{attribute 'no_check'}
//Provides all information of PlcAppSystemInfo plus addtional infos like time stamps from various source and in different formats
//
//PlcAppSystemInfo -> https://infosys.beckhoff.com/english.php?content=../content/1033/globaldatatypes/9007199969559691.html&id=7934476013631172214
//TwimCAT time sources -> https://infosys.beckhoff.com/english.php?content=../content/1033/ethercatsystem/2469114379.html&id=
//
FUNCTION_BLOCK SystemInfo
VAR_OUTPUT CONSTANT
{attribute 'displaymode':='binary'}
	OPTION_US_DATE_FORMAT									:	BYTE := 2#0000_0001; //Enable US date format in time stamp - mm/dd/yy
{attribute 'displaymode':='binary'}
	OPTION_US_TIME_FORMAT									:	BYTE := 2#0000_0010; //Enable time in US format - AM/PM vs 24h
{attribute 'displaymode':='binary'} 
	OPTION_TIME_STR_ADD_MS									:	BYTE := 2#0000_0100; //Add ms to time string 
{attribute 'displaymode':='binary'} 
	OPTION_DISABLE_DEV_IDENT								:	BYTE := 2#0000_1000; //Disable to read device identification during boot up (Call FB_GetDeviceIdentificationEx)
END_VAR                     								
VAR_INPUT                   						
	Enable													:	BOOL := TRUE; //Enable function block
	ResetTrig												:	BOOL := FALSE; //Reset Old boot data fault signal
	RtcSyncCylce											:	DWORD := 60; //in seconds - see documentation for "FB_LocalSystemTime"
	KeepOutputsOnBP 										: 	BOOL := FALSE; //The flag can be set to avoid that the outputs are zero-filled if a breakpoint is reached. The task keeps running. Only the execution of PLC code is interrupted.
{attribute 'displaymode':='binary'}
	Options													:	BYTE := 2#0000_0000; //option constants are alreay predefined, so they can accordingly be passed symbolically to the block 
	DateStrSeperator										:	STRING(1) := '/';
END_VAR
VAR_OUTPUT
//PlcAppSystemInfo and cycle time inforamtion from caller task 
	ObjId													: 	OTCID; //Object ID of the PLC project instance
	AdsPort 												: 	UINT; //ADS port of PLC application 
	TComSrvPtr 												: 	ITComObjectServer; // Pointer to TcCOM Object Server 
	AppName													: 	STRING(63); //TwinCAT generated name containing the port number. 
	ProjectName 											: 	STRING(63); //The name of the PLC project. 
	AppTimestampDT											:	DT; //Date and time of application start 
	AppTimestamp											:	STRING(25);	//Date and time of application start in string format
	TaskIndex												:	INT ; //Task index of SysInfo caller
	TaskCnt													: 	UDINT; //The number of tasks in the actual runtime system
	
	Flags 													: 	DWORD; //Boot flags
	LicensesPending 										: 	BOOL;
	BSODOccured 											: 	BOOL;										
	BootDataLoaded											: 	BOOL;//PERSISTENT variables: LOADED (without error)
	OldBootData												: 	BOOL; //PERSISTENT variables: INVALID (the back-up copy was loaded, since no valid data was present)
	NoBootDataLoaded										:	BOOL; //Error no boot data loaded
//	PersistentStatus 										: 	EPlcPersistentStatus;

	LoggedIn												:	BOOL;
	ShutdownInProgress 										: 	BOOL;	
	OnlineChangeCount										: 	UDINT; //The number of online changes made since the last complete download.
	OnlineChange											:	BOOL; //Online change count changed since last plc cycle

{attribute 'displaymode':='hex'}
	CpuCounter												:	ULINT;
	CycleTime         										: 	UDINT;//Cylce time read from PlcAppSystemInfo in multiples of 100 ns.
	CycleTimeNS         									: 	UDINT;//Cylce time in nanoseconds
	CycleTimeT       										: 	TIME; //Cycle time in time format
	CycleTimeLT       										: 	LTIME; //Cycle time in ltime format
	CycleTimeFloat											:	LREAL;//Cycle time in float format <s.ms>

	DevIdentValid											:	BOOL;
	pDevIdent												:	POINTER TO ST_DeviceIdentificationEx := ADR(InstGetDevIdent.stDevIdent);
	
//General	
	TimezoneId												: 	E_TimeZoneID;
	TimeZoneInfo											:	ST_TimeZoneInformation;
	MonthDays												:	WORD;
	LeapYear												:	BOOL;
	DayOfYear												:	WORD;
	WeekOfYear												:	WORD;
	UtcTimeFT												:	Tc2_Utilities.T_FILETIME; //Current UTC System/TwinCAT time T_FILETIME format, structure representing a 64-bit value with the a number of 100-nanosecond intervals since January 1, 1601 (UTC) (dwLowDateTime : DWORD / dwHighDateTime : DWORD)
//	UtcTimeFT												:	Tc2_Utilities.T_FILETIME64; //Current UTC System/TwinCAT time T_FILETIME format, structure representing a 64-bit value with the a number of 100-nanosecond intervals since January 1, 1601 (UTC) (dwLowDateTime : DWORD / dwHighDateTime : DWORD)
	UtcTimeSTRUCT											:	Tc2_Utilities.TIMESTRUCT; //Current UTC System/TwinCAT time in TIMESTRUCT format
	UtcTimezoneBias											:	DINT;   //Total timezone bias in minutes to UTC 
	TimeDT													:	DATE_AND_TIME;	//Current time in DATE_AND_TIME format: DT#1970-01-01-00:00 -> DT#2106-02-06-06:28:15
//	TimeLDT													:	LDATE_AND_TIME;	//Current time in 64bit LDATE_AND_TIME format: DT#1970-01-01-00:00 -> DT#2262-4-10-23:59:59.99999999
	TimeTOD													:	TOD; //Current time in TOD format, range from TOD#00:00 -> TOD#1193:02:47.295
	TimeFT													:	Tc2_Utilities.T_FILETIME; //Current time in T_FILETIME format, structur representing a 64-bit value with the a number of 100-nanosecond intervals since January 1, 1601 (UTC) (dwLowDateTime : DWORD / dwHighDateTime : DWORD)
//	TimeFT													:	Tc2_Utilities.T_FILETIME64; //Current time in T_FILETIME format, structur representing a 64-bit value with the a number of 100-nanosecond intervals since January 1, 1601 (UTC) (dwLowDateTime : DWORD / dwHighDateTime : DWORD)
	TimeSTRUCT												:	Tc2_Utilities.TIMESTRUCT; //Current time in TIMESTRUCT format
	Datestamp												:	DATE; //D#1970-01-01 -> D#2106-02-06
	DateStr													:	STRING(15);	(* dd.mm.jj or mm.dd.jj *)	
	TimeStr													:	STRING(15);	(* hh:mm:ss.xxx or hh:mm:ss.xxxPM/AM *)
	TimeStamp												:	STRING(25); (* DateStr + TimeStr *)	
	TimeStamp2												:	STRING(25); (* YYYY-MM-DDTHHMMSS for example YYYY-MM-DD_HHMMSS_Name.txt *)
	TimeStamp3												:	STRING(25); (* YYYY-MM-DD-hh:mm:ss.xxx *)
	DateStrISO												:	STRING(15);	(* jj-mm-dd *)
	TimeStrISO												:	STRING(15);	(* hh:mm:ss *)
	TimeStampISO											:	STRING(25);	(* jj-mm-dd'T'hh:mm:ss.xxms *)	
	TimeStampStartup										:	DATE_AND_TIME; //Timestamp of startup
	DCTime													:	Tc2_EtherCAT.T_DCTIME64; //Current TwinCAT distributed clock time in 64-bit T_DCTIME64 format. The smallest unit is a nanosecond.
	DCTimeSTRUCT											:	Tc2_Utilities.TIMESTRUCT;//Current TwinCAT distributed clock time in TIMESTRUCT format
//	SysTimeFT												:	Tc2_Utilities.T_FILETIME64; //Current UTC System/TwinCAT time T_FILETIME format, structure representing a 64-bit value with the a number of 100-nanosecond intervals since January 1, 1601 (UTC) (dwLowDateTime : DWORD / dwHighDateTime : DWORD)
	SysTimeFT												:	Tc2_Utilities.T_FILETIME; //Current UTC System/TwinCAT time T_FILETIME format, structure representing a 64-bit value with the a number of 100-nanosecond intervals since January 1, 1601 (UTC) (dwLowDateTime : DWORD / dwHighDateTime : DWORD)
	SysTimeSTRUCT											:	Tc2_Utilities.TIMESTRUCT; //Current UTC System/TwinCAT time in TIMESTRUCT format
	
END_VAR
VAR
	(* Inst. Get Taskindex *)
	InstGETCURTASKINDEX										: 	GETCURTASKINDEX;
	InstLocalSystemTime										:	FB_LocalSystemTime;
	InstNtSetLocalTime										:	NT_SetLocalTime := (NETID := '', TMOUT := DEFAULT_ADS_TIMEOUT);
	InstTimeZoneInfo										:	FB_GetTimeZoneInformation;
	InstCpuCouter											:	GETCPUCOUNTER;
	InstSystemTime											:	GetSystemTime;
	
	
	InstGetDevIdent											:	FB_GetDeviceIdentificationEx;
	_OnlineChangeCount										: 	UDINT; 
	_sec													:	WORD;
	_hour													:	WORD;
	_day													:	WORD;
	_Init													:	BOOL;
END_VAR

	(* Evaluate the PlcAppSystemInfo and and get sytstem timestamp					*)
	(********************************************************************************)
	
(* Get Current Task Index ************************************************************************)
	IF InstGETCURTASKINDEX.index = 0 then InstGETCURTASKINDEX(index => TaskIndex); END_IF

(* Read System Info Current Task *****************************************************************)	
	(* Get static information and boot error messages *)
	IF TwinCAT_SystemInfoVarList._TaskInfo[InstGETCURTASKINDEX.Index].FirstCycle 
	THEN
		AppTimestampDT										:= TwinCAT_SystemInfoVarList._AppInfo.AppTimestamp;
		AppTimestamp										:= DT_TO_STRING(AppTimestampDT);
		AppTimestamp										:= DELETE(AppTimestamp,3,1);
			
		TaskIndex											:= InstGETCURTASKINDEX.Index;
		TaskCnt 											:= TwinCAT_SystemInfoVarList._AppInfo.TaskCnt;
		
		ObjId												:= TwinCAT_SystemInfoVarList._AppInfo.ObjId;
		AppName												:= TwinCAT_SystemInfoVarList._AppInfo.AppName;	
		ProjectName											:= TwinCAT_SystemInfoVarList._AppInfo.ProjectName;	
		AdsPort												:= TwinCAT_SystemInfoVarList._AppInfo.AdsPort;	
			
		Flags												:= TwinCAT_SystemInfoVarList._AppInfo.Flags;
//		PersistentStatus									:= TwinCAT_SystemInfoVarList._AppInfo.PersistentStatus;
		
		BootDataLoaded										:= TwinCAT_SystemInfoVarList._AppInfo.BootDataLoaded;
		OldBootData											:= TwinCAT_SystemInfoVarList._AppInfo.OldBootData;
		NoBootDataLoaded									:= NOT BootDataLoaded AND NOT OldBootData;
		BSODOccured 										:= TwinCAT_SystemInfoVarList._AppInfo.BSODOccured;
		
		CycleTime         									:= TwinCAT_SystemInfoVarList._TaskInfo[TaskIndex].CycleTime;
		CycleTimeNS         								:= TwinCAT_SystemInfoVarList._TaskInfo[TaskIndex].CycleTime * 100;
		CycleTimeT											:= LREAL_TO_TIME(UDINT_TO_LREAL(CycleTime) * 0.0001 );
		CycleTimeLT											:= TO_LTIME(CycleTimeNS);	
		CycleTimeFloat										:= (UDINT_TO_LREAL(CycleTime) * 0.0001 / 1000.0);	
		
	ELSIF ResetTrig
	THEN
		resetBootInfo();
	ELSIF NOT Enable
	THEN
		RETURN;
	END_IF
	
	OnlineChangeCount										:= TwinCAT_SystemInfoVarList._AppInfo.OnlineChangeCnt;
	OnlineChange											:= _OnlineChangeCount <> OnlineChangeCount;
	_OnlineChangeCount										:= OnlineChangeCount;
	LoggedIn 												:= TwinCAT_SystemInfoVarList._AppInfo.LoggedIn;
	ShutdownInProgress 										:= TwinCAT_SystemInfoVarList._AppInfo.ShutdownInProgress;
	LicensesPending 										:= TwinCAT_SystemInfoVarList._AppInfo.LicensesPending;
	TComSrvPtr												:= TwinCAT_SystemInfoVarList._AppInfo.TComSrvPtr;
	TwinCAT_SystemInfoVarList._AppInfo.KeepOutputsOnBP		:= KeepOutputsOnBP;		

(* CPU System counter ****************************************************************************)
	InstCpuCouter(cpuCntLoDW => CpuCounter);	
	MEMCPY(ADR(CpuCounter) + SIZEOF(InstCpuCouter.cpuCntHiDW),ADR(InstCpuCouter.cpuCntHiDW),SIZEOF(InstCpuCouter.cpuCntHiDW));
	
(* Get device identification structure ***********************************************************)
	InstGetDevIdent(
		bExecute	:= NOT Options.3, 
		tTimeout	:= , 
		sNetId		:= , 
		bBusy		=> , 
		bError		=> , 
		nErrorID	=> , 
		stDevIdent	=> );	
	pDevIdent												:= ADR(InstGetDevIdent.stDevIdent);
	IF NOT InstGetDevIdent.bBusy
	THEN
		DevIdentValid										:= NOT InstGetDevIdent.bError;
		
		IF InstGetDevIdent.bError AND ResetTrig
		THEN
			InstGetDevIdent(bExecute := FALSE);			
		END_IF
	ELSE	
		DevIdentValid										:= FALSE;
	END_IF
	
(* Read timezone information every day time ******************************************************)
	IF Enable AND NOT InstTimeZoneInfo.bExecute
		OR InstTimeZoneInfo.bBusy
	THEN
		InstTimeZoneInfo(
			sNetID	:= , 
			bExecute:= TRUE, 
			tTimeout:= , 
			bBusy	=> , 
			bError	=> , 
			nErrID	=> , 
			tzID	=> TimeZoneId, 
			tzInfo	=> TimeZoneInfo);
		IF NOT InstTimeZoneInfo.bBusy 
		THEN
			CASE TimeZoneId OF 
			eTimeZoneID_Invalid:	UtcTimezoneBias			:= 0;				
			eTimeZoneID_Standard:	UtcTimezoneBias			:= -1 * (TimeZoneInfo.bias);
			eTimeZoneID_Daylight:	UtcTimezoneBias			:= -1 * (TimeZoneInfo.bias + TimeZoneInfo.daylightBias);
			ELSE //eTimeZoneID_Unknown:		
				UtcTimezoneBias								:= 0;	
			END_CASE
		END_IF
	ELSIF NOT Enable AND InstTimeZoneInfo.bExecute 
		OR InstTimeZoneInfo.bError AND ResetTrig
	THEN
		InstTimeZoneInfo(bExecute:= FALSE);
	END_IF
		
(* Actual EtherCAT DC time in DCTIME64 format ****************************************************************)
	DCTime													:= F_GetActualDcTime64();
	DCTimeSTRUCT											:= DCTIME64_TO_SYSTEMTIME(DCTime);

(* Get TwinCAT/system time according to system time zone initialized during TC start ******************************************************)
	InstSystemTime(timeHiDW => UtcTimeFT.dwHighDateTime,timeLoDW => UtcTimeFT.dwLowDateTime );
	SysTimeSTRUCT											:= FILETIME_TO_SYSTEMTIME(UTCTimeFT);	
	
//	SysTimeFT												:= F_GetSystemTime();	 
//	SysTimeSTRUCT											:= FILETIME64_TO_SYSTEMTIME(UTCTimeFT);	 
	
(* evalutate systemtime ************************************************************************)
	InstLocalSystemTime(
		sNetID		:= '',
		bEnable		:= Enable,
		dwCycle		:= SEL(InstNtSetLocalTime.START, RtcSyncCylce, 1), //Short update cylce to read windows time after it was set
		dwopt		:= (* Default *),
		tTimeout	:= (* Default *),
		bValid		=> ,
		systemTime	=> TimeSTRUCT,
		tzID		=> );

(* Get TwinCAT/system time in UTC Filetime format ******************************************************)
	IF InstLocalSystemTime.bValid 
	THEN				
		//Update cyclic
//		TimeFT												:= SYSTEMTIME_TO_FILETIME64(TimeSTRUCT);
		TimeFT												:= SYSTEMTIME_TO_FILETIME(TimeSTRUCT);
		TimeDT 												:= SYSTEMTIME_TO_DT(TimeSTRUCT);
//		TimeLDT												:= SYSTEMTIME_TO_LDT(TimeSTRUCT);	
		TimeStamp3											:= SYSTEMTIME_TO_STRING(TimeSTRUCT);
		TimeTOD												:= SEL(Options.2 ,TO_TOD(TimeDT)  , DWORD_TO_TOD(TO_DWORD(TO_TOD(TimeDT)) + TimeSTRUCT.wMilliseconds));  
		TimeStrISO											:= DELETE(TO_STRING(TimeTOD),4,1);
		TimeStampISO										:= CONCAT(DateStrISO , CONCAT('T',TimeStrISO));
		
		UtcTimeFT											:= F_TranslateFileTimeBias(TimeFT,UtcTimezoneBias,TRUE);
		UtcTimeSTRUCT										:= FILETIME_TO_SYSTEMTIME(UTCTimeFT);	
//		UtcTimeFT											:= F_TranslateFileTime64Bias(TimeFT,UtcTimezoneBias,TRUE);
//		UtcTimeSTRUCT										:= FILETIME64_TO_SYSTEMTIME(UTCTimeFT);	
	
		//Create time format
		IF Options.1
		THEN (* US time format hh.mm.ss AM/PM ***************)
			IF TimeSTRUCT.wHour < 10 
			THEN
				TimeStr 									:= CONCAT('0',WORD_TO_STRING(TimeSTRUCT.wHour));
			ELSIF TimeSTRUCT.wHour > 12 
			THEN
				TimeStr 									:= WORD_TO_STRING(TimeSTRUCT.wHour - 12);
				IF TimeSTRUCT.wHour - 12 < 10
				THEN
					TimeStr									:= CONCAT('0',TimeStr);
				END_IF
			ELSE         									
				TimeStr 									:= WORD_TO_STRING(TimeSTRUCT.wHour);
			END_IF		                                    
		ELSE  (* Time hh.mm.ss.xxms ***************)          
			IF TimeSTRUCT.wHour < 10                        
			THEN                                            
				TimeStr 									:= CONCAT('0',WORD_TO_STRING(TimeSTRUCT.wHour));
			ELSE        									
				TimeStr 									:= WORD_TO_STRING(TimeSTRUCT.wHour);
			END_IF			
		END_IF
		
		TimeStr 											:= CONCAT(TimeStr,':');
		
		IF TimeSTRUCT.wMinute < 10 
		THEN
			TimeStr 										:= CONCAT(TimeStr,CONCAT('0',WORD_TO_STRING(TimeSTRUCT.wMinute)));
		ELSE
			TimeStr 										:= CONCAT(TimeStr,WORD_TO_STRING(TimeSTRUCT.wMinute));
		END_IF
		
		TimeStr 											:= CONCAT(TimeStr,':');
		
		IF TimeSTRUCT.wSecond < 10 
		THEN
			TimeStr 										:= CONCAT(TimeStr,CONCAT('0',WORD_TO_STRING(TimeSTRUCT.wSecond)));
		ELSE        										
			TimeStr 										:= CONCAT(TimeStr,WORD_TO_STRING(TimeSTRUCT.wSecond));
		END_IF  
												
		IF Options.2
		THEN //add ms to timestamp
			TimeStr 										:= CONCAT(TimeStr,'.');
			TimeStr 										:= CONCAT(TimeStr,WORD_TO_STRING(TimeSTRUCT.wMilliseconds));
		END_IF
		
		IF Options.1
		THEN //US time format
			TimeStr 										:= CONCAT(TimeStr,SEL(TimeSTRUCT.wHour > 12,' AM', ' PM'));
		END_IF
		
		(* TimeStamp Format DE: DD.MM.YY-Stunde:Minute:Sekunde.xxx,*)
		TimeStamp 											:= CONCAT(DateStr,'-');
		TimeStamp 											:= CONCAT(TimeStamp,TimeStr);
		
		IF _hour <> TimeSTRUCT.wHour OR NOT _Init
		THEN
			_Hour											:= TimeSTRUCT.wHour;		
			//Create date in US fromat with seperator / ************************************************
			IF Options.0
			THEN (* Date mm/dd/jj ********************)
				IF TimeSTRUCT.wMonth < 10 
				THEN
					DateStr 								:= CONCAT('0',WORD_TO_STRING(TimeSTRUCT.wMonth));
				ELSE        								
					DateStr 								:= WORD_TO_STRING(TimeSTRUCT.wMonth);
				END_IF		                                
				DateStr 									:= CONCAT(DateStr,DateStrSeperator);
				IF TimeSTRUCT.wDay < 10                     
				THEN                                        
					DateStr 								:= CONCAT(DateStr,CONCAT('0',WORD_TO_STRING(TimeSTRUCT.wDay)));
				ELSE        								
					DateStr 								:= CONCAT(DateStr,WORD_TO_STRING(TimeSTRUCT.wDay));
				END_IF                                      
															
				DateStr 									:= CONCAT(DateStr,DateStrSeperator);
				DateStr 									:= CONCAT(DateStr,RIGHT(WORD_TO_STRING(TimeSTRUCT.wYear),2));		
		                                                    
			ELSE (* Date dd.mm.jj ********************)	    
				IF TimeSTRUCT.wDay < 10                     
				THEN                                        
					DateStr 								:= CONCAT('0',WORD_TO_STRING(TimeSTRUCT.wDay));
				ELSE        								
					DateStr 								:= WORD_TO_STRING(TimeSTRUCT.wDay);
				END_IF                                      
				DateStr 									:= CONCAT(DateStr,DateStrSeperator);
				IF TimeSTRUCT.wMonth < 10                   
				THEN                                        
					DateStr 								:= CONCAT(DateStr,CONCAT('0',WORD_TO_STRING(TimeSTRUCT.wMonth)));
				ELSE        								
					DateStr 								:= CONCAT(DateStr,WORD_TO_STRING(TimeSTRUCT.wMonth));
				END_IF                                      
															
				DateStr 									:= CONCAT(DateStr,DateStrSeperator);
				DateStr 									:= CONCAT(DateStr,RIGHT(WORD_TO_STRING(TimeSTRUCT.wYear),2));	
			END_IF      

			DateStrISO										:= DELETE(TO_STRING(TO_DATE(TimeDT)),2,1);
			
			(* information of year *)                       
			MonthDays										:= F_GetMaxMonthDays(TimeSTRUCT.wYear,TimeSTRUCT.wMonth);
			LeapYear										:= F_YearIsLeapYear(TimeSTRUCT.wYear) ;
			WeekOfYear										:= F_GetWeekOfTheYear(TimeDT);
			DayOfYear										:= F_GetDOYOfYearMonthDay(TimeSTRUCT.wYear,TimeSTRUCT.wMonth,TimeSTRUCT.wDay);
			DateStamp										:= TO_DATE(TimeDT);		
			
			IF NOT _INIT AND_THEN TO_DINT(TimeStampStartup) = 0  
			THEN					
				TimeStampStartup							:= SYSTEMTIME_TO_DT(TimeSTRUCT);
			END_IF
			
			IF NOT InstTimeZoneInfo.bBusy THEN InstTimeZoneInfo(bExecute:= FALSE); END_IF

            _INIT											:= TRUE;            
		END_IF //hour
		
		IF _sec <> TimeSTRUCT.wSecond 
		THEN	
			_sec 											:= TimeSTRUCT.wSecond;
														
			(* TimeStamp2 FileName YYYY-MM-DD_HHMMSS *)
			TimeStamp2										:= CONCAT(DateStrISO , '_');
			IF TimeSTRUCT.wHour < 10                    	
			THEN                                        	
				TimeStamp2 									:= CONCAT(TimeStamp2,CONCAT('0',WORD_TO_STRING(TimeSTRUCT.wHour)));
			ELSE           									
				TimeStamp2 									:= CONCAT(TimeStamp2,WORD_TO_STRING(TimeSTRUCT.wHour));
			END_IF                                      	
			IF TimeSTRUCT.wMinute < 10                  	
			THEN                                        	
				TimeStamp2 									:= CONCAT(TimeStamp2,CONCAT('0',WORD_TO_STRING(TimeSTRUCT.wMinute)));
			ELSE           									
				TimeStamp2 									:= CONCAT(TimeStamp2,WORD_TO_STRING(TimeSTRUCT.wMinute));
			END_IF                                      	
			IF TimeSTRUCT.wSecond < 10                  	
			THEN                                        	
				TimeStamp2 									:= CONCAT(TimeStamp2,CONCAT('0',WORD_TO_STRING(TimeSTRUCT.wSecond)));
			ELSE           									
				TimeStamp2 									:= CONCAT(TimeStamp2,WORD_TO_STRING(TimeSTRUCT.wSecond));
			END_IF
		END_IF //second update
													
	END_IF

(* set system time *****************************************************************************)
	InstNtSetLocalTime(
		NETID		:= , 
		TIMESTR		:= , 
		START		:= , // Start by Methode "SetSysTime" 
		TMOUT		:= , 
		BUSY		=> , 
		ERR			=> ); 
	
	IF InstNtSetLocalTime.START AND NOT InstNtSetLocalTime.BUSY
	THEN //Take care that all timestamp get updated after set a new time
		InstNtSetLocalTime.START							:= FALSE;	
		_Init												:= FALSE;								
	END_IF
	
(**************************************************************************************************)

PROPERTY PUBLIC actDCTimeWithTimezoneBias : T_DCTIME64
GET
actDCTimeWithTimezoneBias							:= F_GetActualDcTime64() + (TO_ULINT(UtcTimezoneBias) * 60 * EC_DCTIME_TICKSPERSEC64);
END_GET
END_PROPERTY

PROPERTY PUBLIC optAddmsToTimeString : BOOL
GET
optAddmsToTimeString := Options.2;
END_GET
SET
Options.2 := optAddmsToTimeString;
END_SET
END_PROPERTY

PROPERTY PUBLIC  optDisableReadDeviceIdentification : BOOL
GET
optDisableReadDeviceIdentification := Options.3;
END_GET
SET
Options.3 := optDisableReadDeviceIdentification;
END_SET
END_PROPERTY

PROPERTY PUBLIC optEnableUSDateFormat : BOOL
GET
optEnableUSDateFormat := Options.0;
END_GET
SET
Options.0 := optEnableUSDateFormat;
END_SET
END_PROPERTY

PROPERTY PUBLIC optEnableUSTimeFormat : BOOL
GET
optEnableUSTimeFormat := Options.1;
END_GET
SET
Options.1 := optEnableUSTimeFormat;
END_SET
END_PROPERTY

METHOD PUBLIC resetBootInfo : BOOL  //Return value = TRUE if execution finished
VAR_INPUT
END_VAR
OldBootData 												:= FALSE;
BSODOccured													:= FALSE;
NoBootDataLoaded											:= FALSE;
resetBootInfo												:= TRUE;
END_METHOD

METHOD PUBLIC setSysTime  : BOOL //Return value = TRUE if execution finished
VAR_INPUT
	TimeStruct		: TIMESTRUCT;
END_VAR
InstNtSetLocalTime(
		NETID		:= '', 
		TIMESTR		:= TimeStruct, 
		START		:= NOT InstNtSetLocalTime.START AND TimeStruct.wYear > 2000 
						AND TimeStruct.wDay > 0 AND TimeStruct.wMonth	< 32	
						AND TimeStruct.wMonth > 0 AND TimeStruct.wMonth	< 13	
						AND TimeStruct.wHour >= 0 AND TimeStruct.wHour	< 24	
						AND TimeStruct.wMinute >= 0 AND TimeStruct.wMinute < 60
						AND TimeStruct.wSecond >= 0 AND TimeStruct.wSecond < 60				
						OR InstNtSetLocalTime.BUSY, 
		TMOUT		:= , 
		BUSY		=> , 
		ERR			=> , 
		ERRID		=> );
		
setSysTime													:= InstNtSetLocalTime.BUSY;
END_METHOD

END_FUNCTION_BLOCK
